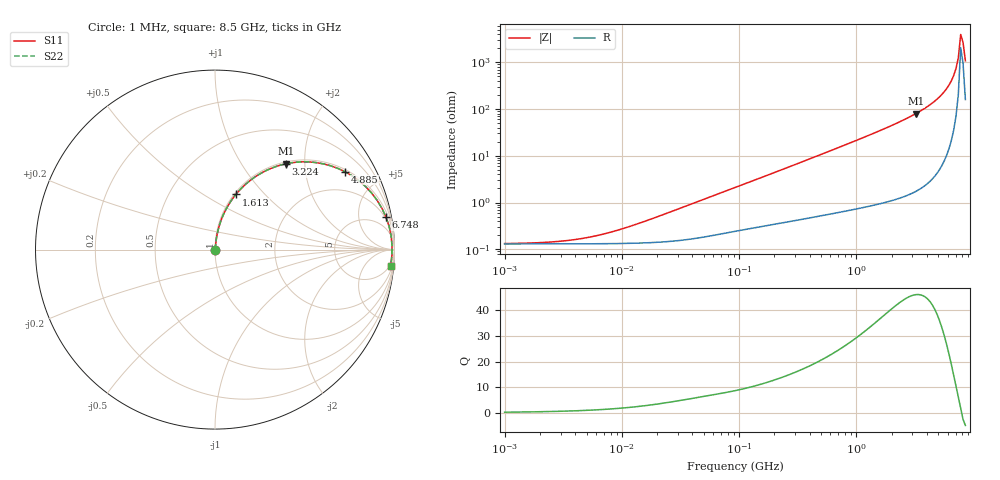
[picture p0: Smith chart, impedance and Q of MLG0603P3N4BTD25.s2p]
! S-Parameter Data Generated by TDK Corporation
! Copyright(C) 2025 TDK Corporation.
! All Rights Reserved.
! TDK P/N: MLG0603P3N4BTD25 (SMD / SMT Inductor (Coil))
! Property: L=3.4nH at 500MHz
! Size(LxWxT): 0.6x0.3x0.3mm
! Model Type: s2p (Touchstone File Format Version 1.0)
! Frequency: DC=Yes Start=1MHz Stop=8500MHz 198points Log-sweep
! Model Generated on Feb. 6, 2025
! Terms and conditions regarding TDK Simulation Models:
! 1)This simulation model is being provided solely for informational
!  purposes. Please refer to the specifications of the products in
!  terms of detailed characteristics of such products.
! 2)In no event shall TDK Corporation of any of its subsidiaries be
!  liable for any loss or damage arising, directly or indirectly,
!  from any information contained in this simulation model, including,
!  but not limited to loss or damages arising from any inaccuracies,
!  omissions or errors in connection with such information.
! 3)Any and all copyrights on this simulation model are owned by
!  TDK Corporation.  Duplication or redistribution of this simulation
!  model without prior written permission from TDK Corporation
!  is prohibited.
! 4)This simulation model is subject to any modification or change
!  without any prior notice.
! 5)Neither TDK Corporation nor any of its subsidiaries shall make any
!  warranty, express or implied, including but not limited to the
!  correctness, implied warranties of merchantability and fitness for
!  a particular purpose with respect to this simulation models.
! 6)The use of this simulation model shall be deemed to have consented
!  to the terms and conditions hereof.
! Port Assignments:
!  1 ---@@@--- 2
! Applicable Conditions:
!  Temperature = 25 degC
!  DC Bias Current = 0 A
!  Small Signal Operation
# Hz S MA R 50
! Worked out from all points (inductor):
!   197 points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, 1 MHz to 8.5 GHz, reference 50 ohm
!   read as one part in series: L = 3.76 nH near 18.32 MHz
!   highest Q = 46.2 at 3.224 GHz (marker M1), where L = 3.96 nH
!   self-resonance near 7.75 GHz
!   S11 on the Smith chart (normalised r, x): 1 MHz: 1.00, +0.00; 1.613 GHz: 1.02, +0.70; 3.224 GHz: 1.03, +1.60; 4.885 GHz: 1.09, +3.28; 6.748 GHz: 2, +10; 8.5 GHz: 4, -21
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1000000  0.00132 10.4  0.9987 -0.0  0.9987 -0.0  0.00132 10.4
2403882  0.00142 23.7  0.9987 -0.0  0.9987 -0.0  0.00142 23.7
4587603  0.0017 39.8  0.9987 -0.1  0.9987 -0.1  0.0017 39.8
9168677  0.002546 58.6  0.9987 -0.1  0.9987 -0.1  0.002546 58.6
2.10461e7  0.005169 73.8  0.9986 -0.3  0.9986 -0.3  0.005169 73.8
9.219544e7  0.02088 82.2  0.9974 -1.2  0.9974 -1.2  0.02088 82.2
4.229561e8  0.08994 81.8  0.9912 -5.2  0.9912 -5.2  0.08994 81.8
8.453103e8  0.1762 77.7  0.9778 -10.1  0.9778 -10.1  0.1762 77.7
1.613203e9  0.3288 69.3  0.9356 -19.2  0.9356 -19.2  0.3288 69.3
1.940355e9  0.3917 65.5  0.9104 -23.0  0.9104 -23.0  0.3917 65.5
2.559585e9  0.5059 58.3  0.8513 -30.4  0.8513 -30.4  0.5059 58.3
3.224109e9  0.6194 50.5  0.7718 -38.3  0.7718 -38.3  0.6194 50.5
4.061159e9  0.7446 40.6  0.651 -48.1  0.651 -48.1  0.7446 40.6
4.884749e9  0.8438 31.0  0.5151 -57.5  0.5151 -57.5  0.8438 31.0
5.87536e9  0.9276 19.9  0.3404 -68.0  0.3404 -68.0  0.9276 19.9
6.44363e9  0.9583 13.9  0.2399 -73.1  0.2399 -73.1  0.9583 13.9
6.748056e9  0.9698 10.8  0.187 -75.4  0.187 -75.4  0.9698 10.8
7.066863e9  0.9785 7.6  0.133 -76.9  0.133 -76.9  0.9785 7.6
7.400733e9  0.9842 4.4  0.07821 -76.1  0.07821 -76.1  0.9842 4.4
7.750377e9  0.9868 1.2  0.02502 -57.4  0.02502 -57.4  0.9868 1.2
8.116539e9  0.9862 -2.0  0.03701 67.0  0.03701 67.0  0.9862 -2.0
8.5e9  0.9824 -5.2  0.09122 76.3  0.09122 76.3  0.9824 -5.2
